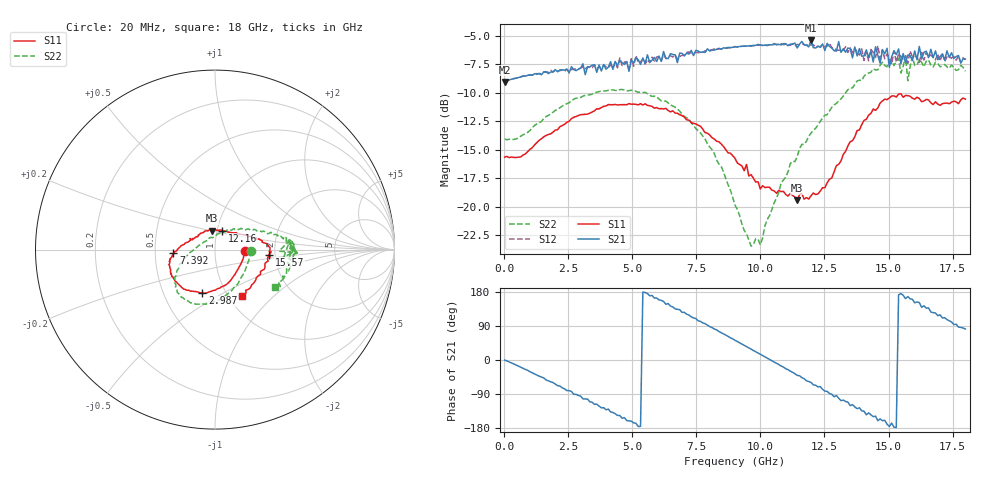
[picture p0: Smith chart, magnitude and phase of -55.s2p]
!Agilent Technologies,N5230A,US43500223,A.07.50.48
!Agilent N5230A: A.07.50.48
!Date: Sunday, January 10, 2016 13:44:22
!Correction: S11(Full 2 Port(1,2))
!S21(Full 2 Port(1,2))
!S12(Full 2 Port(1,2))
!S22(Full 2 Port(1,2))
!S2P File: Measurements: S11, S21, S12, S22:
# Hz S  dB  R 50
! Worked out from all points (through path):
!   201 points, 20 MHz to 18 GHz, reference 50 ohm
!   highest |S21| = -5.39 dB at 11.98 GHz (marker M1); lowest = -9.0 dB at 20 MHz (marker M2)
!   group delay of S21, straight-line fit = 100 ps
!   lowest |S11| = -19.4 dB at 11.44 GHz (marker M3), VSWR 1.24, Z = 47.5 + j10.1 ohm
!   |S11| at or under -10 dB: start of sweep to end of sweep
!   |S22| runs from -23.5 to -6.7 dB; largest |S21 - S12| = 0.097
!   S11 on the Smith chart (normalised r, x): 20 MHz: 1.39, -0.02; 2.987 GHz: 0.78, -0.40; 7.392 GHz: 0.62, -0.03; 12.16 GHz: 1.06, +0.23; 15.57 GHz: 1.86, -0.11; 18 GHz: 1.16, -0.65
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2e7  -15.65 -2.0  -9.04 -0.3  -9.01 -0.4  -14.06 -1.7
1.5483e9  -13.86 -70.4  -8.15 -47.4  -8.18 -48.1  -12.27 -66.7
2.9867e9  -11.92 -106.3  -7.83 -95.4  -7.82 -96.1  -10.40 -96.9
3.0766e9  -11.91 -108.3  -7.44 -102.5  -7.70 -101.0  -10.30 -98.6
4.9645e9  -11.00 -142.6  -7.09 -161.3  -6.99 -165.8  -9.77 -125.3
6.0433e9  -11.40 -158.9  -6.77 158.6  -6.81 155.8  -10.55 -137.1
7.3918e9  -12.68 -175.2  -6.73 110.9  -6.55 110.1  -12.86 -153.0
9.01e9  -15.77 165.8  -5.96 52.0  -5.92 50.7  -19.88 172.6
9.9989e9  -18.45 142.8  -5.80 14.7  -5.81 13.4  -23.37 101.1
1.14373e10  -19.45 98.1  -6.05 -40.6  -5.74 -40.9  -15.61 41.7
1.19767e10  -19.05 76.8  -5.39 -59.2  -5.80 -61.5  -13.55 32.6
1.20666e10  -18.81 72.0  -6.02 -65.5  -5.76 -65.2  -13.27 32.2
1.21565e10  -18.94 68.9  -6.06 -66.7  -6.01 -69.3  -13.12 30.9
1.30555e10  -16.28 35.0  -5.50 -100.9  -6.25 -102.0  -10.72 20.7
1.41343e10  -12.33 13.4  -6.21 -144.7  -6.41 -141.9  -8.33 9.2
1.48535e10  -10.56 4.2  -6.55 -159.1  -7.01 -170.9  -7.60 4.5
1.50333e10  -10.45 3.4  -7.75 -175.5  -6.99 -176.2  -7.11 4.0
1.51232e10  -10.28 2.1  -6.82 -166.4  -7.48 -174.3  -7.19 -1.1
1.55727e10  -10.39 -5.3  -6.55 170.8  -7.13 170.1  -7.69 4.9
1.6202e10  -10.51 -12.9  -5.92 151.5  -7.32 146.0  -7.04 -2.3
1.66515e10  -10.87 -24.1  -6.16 126.7  -6.68 130.5  -7.55 -11.3
1.8e10  -10.55 -59.8  -7.04 81.7  -7.09 76.7  -8.10 -32.0
